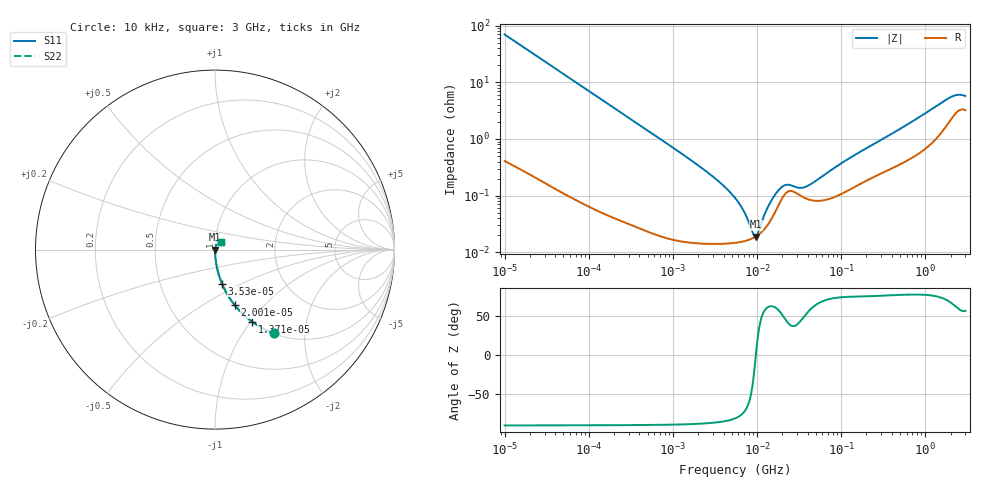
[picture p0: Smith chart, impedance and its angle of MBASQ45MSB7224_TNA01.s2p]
! MBASQ45MSB7224_TNA01  S-PARAMETER MODEL  ( Standard Model )
! Model Generated by TAIYO YUDEN Corporation (http://www.ty-top.com)
! Version 1.0
! TAIYO YUDEN Control No. 220601
! Copyright(c) 2013 TAIYO YUDEN CO.,LTD. All Rights Reserved.
! Product Description (link to TY-COMPAS)
! https://ds.yuden.co.jp/TYCOMPAS/or/detail?pn=MBASQ45MSB7224KTNA01&u=M
! Products Name : Multilayer Ceramic Capacitors
! Characteristics :
!  Capacitance : 0.22 [uF] , Rated Voltage : 250 [V] , TCC : X7R
!  Case Size : 4.5 x 3.2 / 0.177 x 0.126 [mm/inch] , Thickness : 2.5 / 0.098 [mm/inch]
!  (Conditions: Temperature = 25 [degC] , DC Bias Voltage = 0 [V])
! External Node Assignments :
!  1  o---| |---o  2
! GND o---------o GND
! Frequency Range : 10kHz  -  3GHz  [ 401 STEP ]
# MHZ S RI R 50
! Freq[MHz].  S11 Real  S11 Imag  S21 Real  S21 Imag  S12 Real  S12 Imag  S22 Real  S22 Imag
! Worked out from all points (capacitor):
!   401 points, 10 kHz to 3 GHz, reference 50 ohm
!   read as one part in series: C = 229 nF near 10.65 kHz
!   lowest |Z| = 19 mohm at 9.661 MHz (marker M1)
!   series resonance near 9.694 MHz, so ESL is about 1.2 nH
!   S11 on the Smith chart (normalised r, x): 10 kHz: 1.01, -1.39; 13.71 kHz: 1.01, -1.02; 20.01 kHz: 1.00, -0.70; 35.3 kHz: 1.00, -0.40; 3 GHz: 1.06, +0.09
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0.01  0.3269 -0.4661  0.6731 0.4661  0.6731 0.4661  0.3269 -0.4661
0.013707  0.2065 -0.4017  0.7935 0.4017  0.7935 0.4017  0.2065 -0.4017
0.02001  0.1099 -0.3094  0.8901 0.3094  0.8901 0.3094  0.1099 -0.3094
0.035295  0.039 -0.19  0.961 0.19  0.961 0.19  0.039 -0.19
0.082683  0.00787 -0.0841  0.9921 0.0841  0.9921 0.0841  0.00787 -0.0841
0.683653  0.000302 -0.0103  0.9997 0.0103  0.9997 0.0103  0.000302 -0.0103
2.824956  0.000146 -0.00232  0.9999 0.00232  0.9999 0.00232  0.000146 -0.00232
5.477226  0.000148 -0.000904  0.9999 0.000904  0.9999 0.000904  0.000148 -0.000904
7.048603  0.000158 -0.000493  0.9998 0.000493  0.9998 0.000493  0.000158 -0.000493
9.070798  0.00018 -0.000103  0.9998 0.000103  0.9998 0.000103  0.00018 -0.000103
9.6612  0.00019 -5.23e-06  0.9998 5.23e-06  0.9998 5.23e-06  0.00019 -5.23e-06
10.29003  0.000202 9.43e-05  0.9998 -9.43e-05  0.9998 -9.43e-05  0.000202 9.43e-05
14.10408  0.000342 0.000632  0.9997 -0.000632  0.9997 -0.000632  0.000342 0.000632
19.33182  0.000834 0.00111  0.9992 -0.00111  0.9992 -0.00111  0.000834 0.00111
23.35767  0.00118 0.00102  0.9988 -0.00102  0.9988 -0.00102  0.00118 0.00102
34.09912  0.00097 0.000972  0.999 -0.000972  0.999 -0.000972  0.00097 0.000972
45.28751  0.000827 0.00143  0.9992 -0.00143  0.9992 -0.00143  0.000827 0.00143
112.9977  0.00118 0.00398  0.9988 -0.00398  0.9988 -0.00398  0.00118 0.00398
374.4521  0.003 0.0112  0.997 -0.0112  0.997 -0.0112  0.003 0.0112
1929.399  0.0219 0.047  0.9781 -0.047  0.9781 -0.047  0.0219 0.047
2405.867  0.0317 0.0487  0.9683 -0.0487  0.9683 -0.0487  0.0317 0.0487
3000  0.0331 0.0445  0.9669 -0.0445  0.9669 -0.0445  0.0331 0.0445
